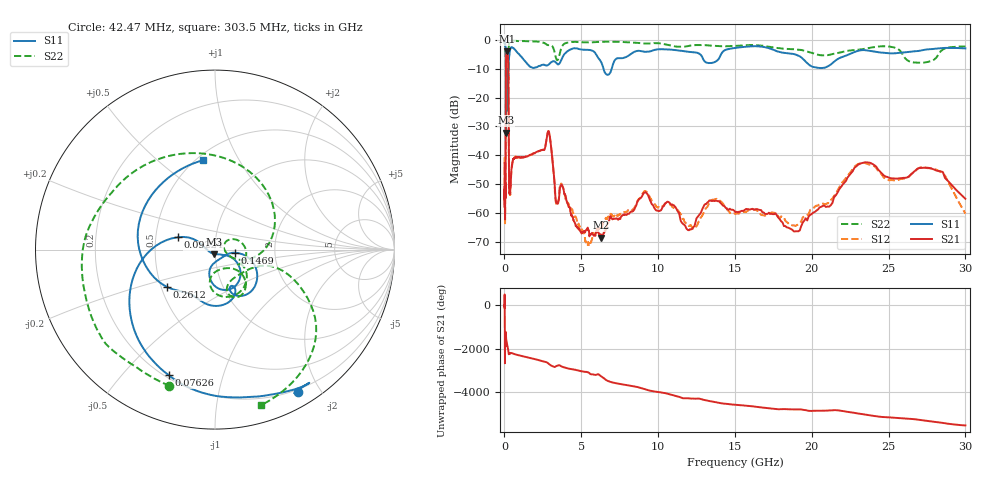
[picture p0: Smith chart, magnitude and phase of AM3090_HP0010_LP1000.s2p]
! Date/Time: Thu, Feb 28, 2019 1:55 PM
! Network Analyzer: Agilent Technologies E8364B Rev: A.07.50.67
! Sweep from 0.010 to 30.000 GHz, 1601 Points, Sweep Type: LOG
! Power Supply: 5.022 V, 0.002 A
# Hz S DB R 50
!freq MagS11 AngS11 MagS21 AngS21 MagS12 AngS12 MagS22 AngS22
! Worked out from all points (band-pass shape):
!   1601 points, 10 MHz to 30 GHz, reference 50 ohm
!   highest |S21| = -3.88 dB at 148.4 MHz (marker M1); lowest = -68.6 dB at 6.296 GHz (marker M2)
!   |S21| within 3 dB of the highest: 101.3 MHz to 238.7 MHz (137.4 MHz wide, 80.8 % of centre)
!   lowest |S11| = -32.1 dB at 99.92 MHz (marker M3), VSWR 1.05, Z = 49.4 - j2.39 ohm
!   |S11| at or under -10 dB: 90.63 MHz to 257.7 MHz (167.1 MHz wide, 95.9 % of centre); 6.451 GHz to 6.98 GHz (529 MHz wide, 7.88 % of centre)
!   |S22| runs from -25.9 to -0.1 dB; largest |S21 - S12| = 0.014
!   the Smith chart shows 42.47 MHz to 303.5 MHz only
!   S11 on the Smith chart (normalised r, x): 42.47 MHz: 0.17, -1.73; 76.26 MHz: 0.21, -0.68; 92.24 MHz: 0.65, +0.09; 146.9 MHz: 1.25, -0.05; 261.2 MHz: 0.54, -0.25; 303.5 MHz: 0.54, +0.72
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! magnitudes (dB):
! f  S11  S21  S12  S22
! 10 MHz  -0.3  -42.7  -40.7  -0.6
! 38.04 MHz  -0.5  -61.3  -61.5  -1.5
! 42.47 MHz  -0.8  -61.4  -59.5  -1.9
! 76.26 MHz  -2.5  -44.8  -46.1  -4.7
! 92.24 MHz  -13.2  -14.0  -14.1  -12.0
! 99.92 MHz  -32.1  -7.4  -7.4  -25.0
! 116.1 MHz  -12.7  -4.9  -4.9  -16.9
! 144.7 MHz  -21.5  -3.9  -3.9  -16.4
! 146.9 MHz  -18.9  -3.9  -3.9  -16.0
! 148.4 MHz  -17.4  -3.9  -3.8  -15.7
! 261.2 MHz  -9.4  -15.2  -15.1  -9.7
! 303.5 MHz  -6.0  -50.5  -50.8  -0.9
! 550.5 MHz  -2.7  -41.5  -41.9  -0.2
! 2.084 GHz  -9.5  -38.8  -39.0  -0.5
! 2.884 GHz  -8.5  -31.7  -31.7  -1.7
! 3.419 GHz  -8.2  -56.8  -57.5  -7.0
! 5.446 GHz  -3.4  -66.1  -70.1  -0.8
! 6.296 GHz  -7.6  -68.6  -65.6  -0.6
! 7.926 GHz  -5.9  -60.7  -59.8  -0.7
! 18.93 GHz  -5.0  -66.4  -64.5  -3.2
! 23.48 GHz  -3.5  -42.4  -42.7  -3.0
! 30 GHz  -2.9  -55.1  -60.2  -2.2
